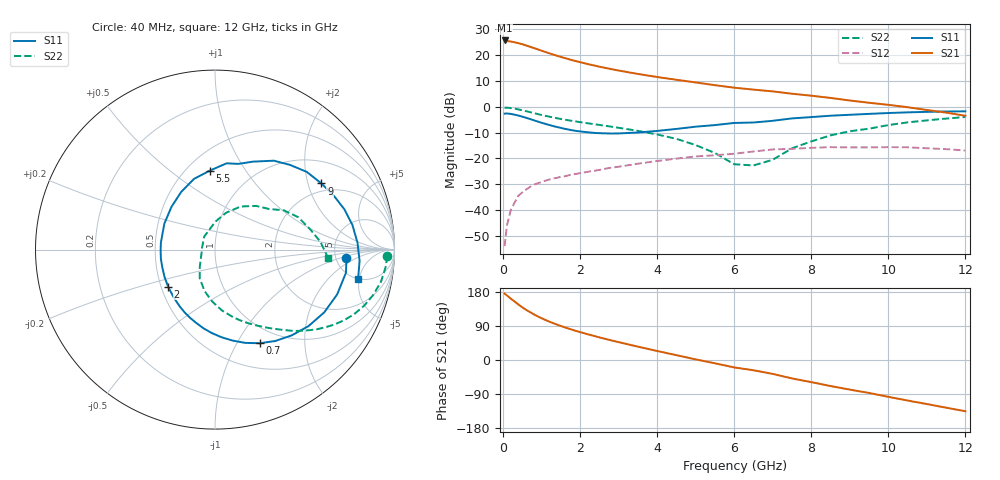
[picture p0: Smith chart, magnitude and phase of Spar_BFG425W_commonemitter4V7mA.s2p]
! Filename: 47bfg425.001
! BFG425W Field C1
! V1=8.277E-001V,V2=4.000E+000V, I1=7.557E-005A, I2=7.010E-003A
# GHz  S  MA  R 50
!  S11  S21  S12  S22
!Freq(GHz)  Mag  Ang  Mag  Ang  Mag  Ang  Mag  Ang
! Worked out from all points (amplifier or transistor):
!   44 points, 40 MHz to 12 GHz, reference 50 ohm
!   highest |S21| = 25.6 dB at 40 MHz (marker M1)
!   |S21| within 3 dB of that: start of sweep to 811.3 MHz
!   unconditionally stable (mu >= 1): start of sweep to 41.25 MHz; 2.166 GHz to end of sweep
!   at 700 MHz: K = 0.45, MSG = 27.1 dB, |S12| = -31.1 dB
!   at 2.4 GHz: K = 1.06, MAG = 18.7 dB, |S12| = -24.7 dB
!   at 12 GHz: K = 1.44, MAG = 2.8 dB, |S12| = -17.0 dB
!   S11 on the Smith chart (normalised r, x): 40 MHz: 6.24, -1.30; 700 MHz: 0.80, -1.25; 2 GHz: 0.54, -0.25; 5.5 GHz: 0.64, +0.70; 9 GHz: 1.70, +2.44; 12 GHz: 4.92, -4.83
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0.04  0.734 -3.8  19.16 175.2  0.002 40.5  0.959 -2.1
0.2  0.725 -20.1  18.26 162.0  0.01 71.8  0.942 -10.9
0.3  0.702 -29.8  17.66 154.2  0.014 69.4  0.917 -16.0
0.4  0.673 -39.3  16.97 146.4  0.019 65.4  0.887 -20.7
0.5  0.641 -48.2  16.2 138.9  0.022 62.2  0.854 -25.0
0.6  0.61 -56.6  15.32 132.3  0.025 58.9  0.819 -28.8
0.7  0.578 -64.5  14.47 126.3  0.028 55.9  0.785 -32.2
0.8  0.546 -72.1  13.66 120.5  0.031 53.5  0.751 -35.2
1  0.489 -85.9  12.14 110.2  0.035 49.6  0.692 -40.5
1.3  0.422 -104.2  10.23 97.2  0.041 45.3  0.619 -46.9
1.6  0.374 -121.2  8.756 86.2  0.045 42.3  0.562 -52.1
2  0.333 -141.6  7.272 73.6  0.052 39.3  0.503 -58.6
2.2  0.32 -151.5  6.69 67.9  0.055 37.9  0.478 -61.8
3  0.304 172.5  5.015 47.1  0.069 31.7  0.391 -74.8
3.5  0.317 152.9  4.312 35.2  0.079 27.0  0.341 -83.5
4.5  0.372 120.6  3.322 12.8  0.099 15.3  0.239 -103.9
5.5  0.441 93.8  2.611 -8.7  0.115 1.6  0.127 -131.8
6.5  0.495 74.8  2.143 -27.1  0.136 -8.6  0.073 172.9
8.5  0.67 40.2  1.479 -68.7  0.165 -45.0  0.279 59.4
9  0.698 31.9  1.32 -78.2  0.163 -53.3  0.335 46.6
10.5  0.778 10.1  0.978 -107.0  0.164 -80.7  0.498 21.3
12  0.814 -11.7  0.668 -135.2  0.142 -111.6  0.633 -4.5
